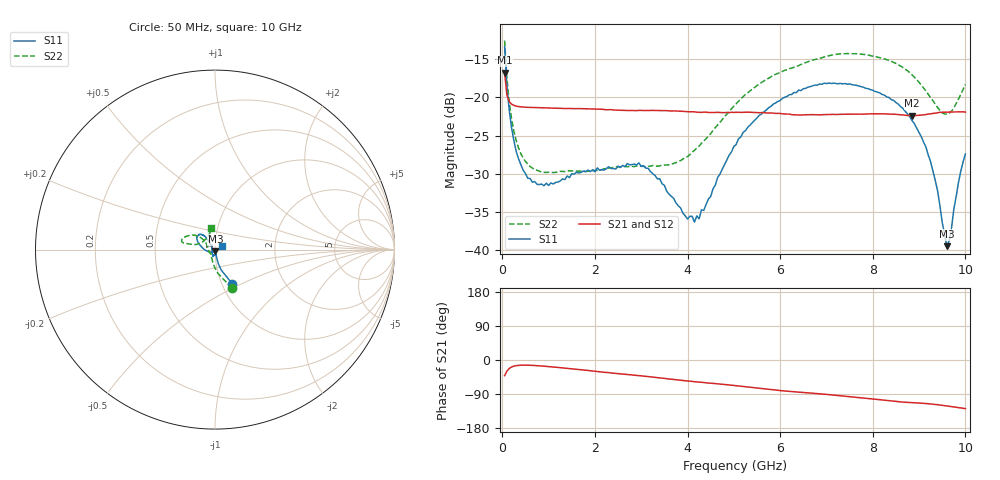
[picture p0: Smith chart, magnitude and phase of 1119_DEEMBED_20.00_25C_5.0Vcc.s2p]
!Hittite Microwave Corp.
!Digital Attenuator/PhaseShifter Rev 1.4.0
!Filename: C:\DATA\DATA\1119_DEEMBED_20.00_25C_5.0Vcc.s2p
!VNA ID: Agilent Technologies,N5224A,MY51441122,A.10.45.03
!Device type:
!2 Port Calibration.
!Temp(C): 25
!Lot Number:
!Serial Number:
!Operator:
!Misc:
!Attenuator:  20.000
# GHZ S DB R 50.0
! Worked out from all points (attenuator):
!   200 points, 50 MHz to 10 GHz, reference 50 ohm
!   highest |S21| = -16.80 dB at 50 MHz (marker M1); lowest = -22.4 dB at 8.85 GHz (marker M2)
!   lowest |S11| = -39.4 dB at 9.6 GHz (marker M3), VSWR 1.02, Z = 50.2 - j1.04 ohm
!   |S11| at or under -10 dB: start of sweep to end of sweep
!   |S22| runs from -29.8 to -12.6 dB; largest |S21 - S12| = 0.00027
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0.05  -13.39 -63.2  -16.80 -41.2  -16.81 -41.3  -12.59 -66.4
0.1  -18.55 -73.2  -19.74 -29.3  -19.73 -29.3  -17.55 -83.3
0.2  -23.99 -77.6  -20.90 -18.4  -20.90 -18.4  -22.84 -100.0
0.35  -28.03 -77.8  -21.22 -14.2  -21.21 -14.1  -26.62 -113.9
0.55  -30.57 -78.8  -21.32 -13.7  -21.32 -13.7  -28.71 -125.5
1  -31.52 -86.4  -21.41 -17.3  -21.40 -17.4  -29.79 -135.9
1.75  -29.63 -102.0  -21.50 -26.3  -21.50 -26.3  -29.64 -139.3
2.95  -28.57 -109.8  -21.72 -41.2  -21.73 -41.2  -29.01 -158.4
3.4  -30.64 -121.8  -21.74 -47.1  -21.75 -47.2  -28.95 -171.7
4.15  -36.30 -177.5  -21.91 -57.3  -21.92 -57.3  -26.93 157.7
5.05  -26.17 126.8  -21.97 -67.8  -21.99 -67.8  -20.84 139.7
5.75  -21.37 127.1  -22.06 -77.2  -22.07 -77.3  -17.52 144.0
6.7  -18.52 134.9  -22.27 -87.7  -22.28 -87.7  -15.16 154.6
7.5  -18.26 146.1  -22.21 -96.8  -22.22 -96.8  -14.31 163.9
8.35  -20.04 158.2  -22.20 -107.3  -22.21 -107.3  -15.20 168.0
8.85  -23.06 171.7  -22.40 -112.6  -22.41 -112.6  -17.09 167.6
9.25  -28.45 -162.6  -22.17 -116.0  -22.18 -116.0  -20.06 161.8
9.400001  -32.24 -145.1  -22.02 -117.9  -22.04 -117.9  -21.34 153.3
9.6  -39.44 -76.2  -21.94 -121.4  -21.95 -121.4  -22.20 132.8
9.7  -37.10 -24.3  -21.92 -123.0  -21.94 -123.0  -21.84 121.0
9.85  -31.14 16.3  -21.92 -125.6  -21.92 -125.6  -20.24 107.4
10  -27.41 30.5  -21.94 -128.3  -21.94 -128.3  -18.32 99.5
